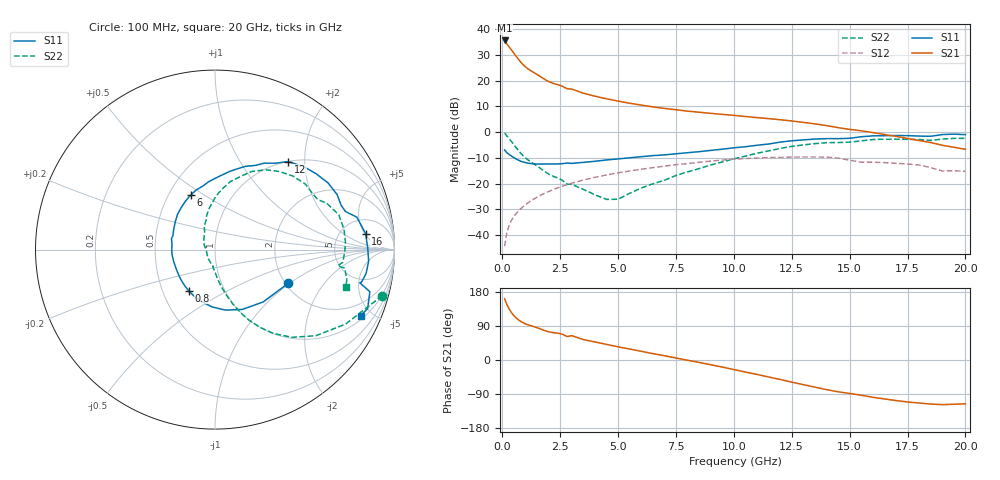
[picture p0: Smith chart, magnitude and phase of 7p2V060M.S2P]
! Infineon Technologies  Discrete & RF Semiconductors
! bfp620
! VCE =  2.0 V,  IC =  60 mA
! Common Emitter S-Parameters:  Sep 2002
# GHz  S  MA  R  50
!  f  S11  S21  S12  S22
! GHz  MAG  ANG  MAG  ANG  MAG  ANG  MAG  ANG
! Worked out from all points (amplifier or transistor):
!   59 points, 100 MHz to 20 GHz, reference 50 ohm
!   highest |S21| = 35.6 dB at 100 MHz (marker M1)
!   |S21| within 3 dB of that: start of sweep to 337.5 MHz
!   unconditionally stable (mu >= 1): 2.623 GHz to 9.845 GHz; 17.18 GHz to end of sweep
!   at 1 GHz: K = 0.87, MSG = 26.8 dB, |S12| = -28.2 dB
!   at 5.5 GHz: K = 1.04, MAG = 12.0 dB, |S12| = -15.1 dB
!   at 20 GHz: K = 1.26, MAG = 1.2 dB, |S12| = -15.2 dB
!   S11 on the Smith chart (normalised r, x): 100 MHz: 2.07, -0.97; 800 MHz: 0.68, -0.33; 6 GHz: 0.64, +0.44; 12 GHz: 1.00, +1.66; 16 GHz: 8.48, +5.28; 20 GHz: 1.20, -4.33
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0.1  0.4487 -24.8  59.98 161.5  0.0061 82.4  0.9664 -15.4
0.2  0.3965 -47.3  51.17 146.1  0.0113 73.9  0.8377 -29.7
0.3  0.3666 -65.4  44.66 134.0  0.0157 70.8  0.7387 -40.5
0.4  0.3421 -80.2  39.04 124.6  0.0195 69.0  0.6506 -48.7
0.5  0.3197 -92.9  33.98 117.1  0.023 67.9  0.5701 -55.1
0.6  0.3002 -104.1  29.53 111.0  0.0263 67.1  0.4984 -60.1
0.7  0.2843 -114.1  25.77 105.9  0.0294 66.5  0.4372 -64.2
0.8  0.272 -122.7  22.71 101.7  0.0326 66.1  0.3869 -67.4
1  0.2555 -136.3  18.45 95.4  0.0388 65.3  0.3152 -72.1
1.2  0.246 -146.2  15.86 91.1  0.0451 64.5  0.2697 -75.2
1.9  0.2404 -172.7  10.13 76.3  0.0671 60.2  0.1638 -85.0
2.8  0.2505 165.7  6.923 61.8  0.0954 53.0  0.0977 -96.9
3  0.2468 161.9  6.852 64.3  0.1017 51.2  0.0965 -95.6
3.5  0.2583 152.5  5.67 53.9  0.1172 46.6  0.0773 -108.3
6  0.3327 114.1  3.341 22.9  0.19 22.6  0.0819 139.6
7  0.3605 100.8  2.878 11.4  0.2181 12.9  0.1158 119.9
10.5  0.5193 64.5  2.006 -31.9  0.3072 -26.6  0.3419 83.0
12  0.6383 50.2  1.735 -51.3  0.3208 -44.3  0.4813 64.8
13.5  0.7315 30.5  1.442 -71.6  0.3276 -63.2  0.5967 43.4
16  0.8438 6.1  0.981 -98.4  0.2606 -87.1  0.7165 15.8
17  0.8585 -4.3  0.827 -107.0  0.2478 -95.1  0.728 3.5
20  0.8923 -24.3  0.464 -115.7  0.1732 -104.6  0.7566 -15.8
